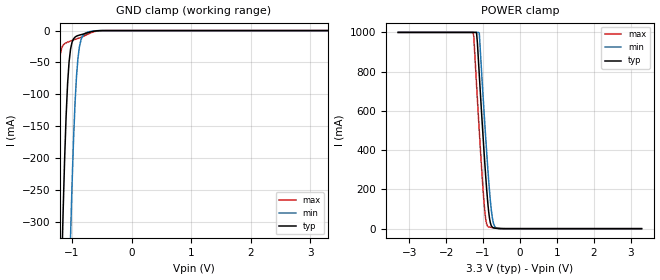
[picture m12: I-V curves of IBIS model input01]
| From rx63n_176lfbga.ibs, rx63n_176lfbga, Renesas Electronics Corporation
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[Model]   input01
Model_type   Input
Vinl  =   0.660V
Vinh  =   2.640V
| variable   typ   min   max
C_comp   3.640pF   3.640pF   3.640pF
| variable   typ   min   max
[Temperature Range]   45.000   105.000   -40.000
| variable   typ   min   max
[Voltage Range]   3.300V   3.000V   3.600V
| variable   typ   min   max
[POWER Clamp Reference] 3.300V   3.000V   3.600V
| variable   typ   min   max
[GND Clamp Reference]   0.000V   0.000V   0.000V
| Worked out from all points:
|   GND clamp passes 1 mA (typ) near -0.63 V on its own axis
|   POWER clamp passes 1 mA (typ) near -0.58 V on its own axis
[GND Clamp]
| input01 GNDClamp rx631_rx63n
| Thu Mar 22 17:15:49 2012
| voltage   I(typ)   I(min)   I(max)
-3.3V     -1A        -1A        -1A
-1.325V   -1A        -1A        -369.2mA
-1.3V     -928.6mA   -1A        -269.7mA
-1.25V    -694.8mA   -1A        -112.6mA
-1.175V   -376mA     -953.3mA   -27.44mA
-1.15V    -283.8mA   -837.7mA   -22.69mA
-1.075V   -83.42mA   -512.2mA   -18.16mA
-1.025V   -28.94mA   -323mA     -16.39mA
-925mV    -8.707mA   -71.38mA   -13.1mA
-850mV    -6.468mA   -14.65mA   -10.64mA
-675mV    -1.81mA    -1.082mA   -3.186mA
3.3V      0A         0A         0A
[POWER Clamp]
| input01 PWRClamp rx631_rx63n
| Thu Mar 22 17:15:49 2012
| voltage   I(typ)   I(min)   I(max)
-3.3V     1A         1A         1A
-1.275V   1A         1A         1A
-1.25V    1A         1A         982.1mA
-1.175V   1A         1A         736.6mA
-1.1V     784.3mA    995.9mA    498mA
-1V       476.2mA    683.1mA    204.7mA
-950mV    332.1mA    533mA      87.52mA
-875mV    143.3mA    321.7mA    12.76mA
-825mV    55.42mA    197.2mA    7.873mA
-750mV    8.119mA    59.94mA    5.513mA
-625mV    1.619mA    2.607mA    2.132mA
3.3V      0A         0A         0A
